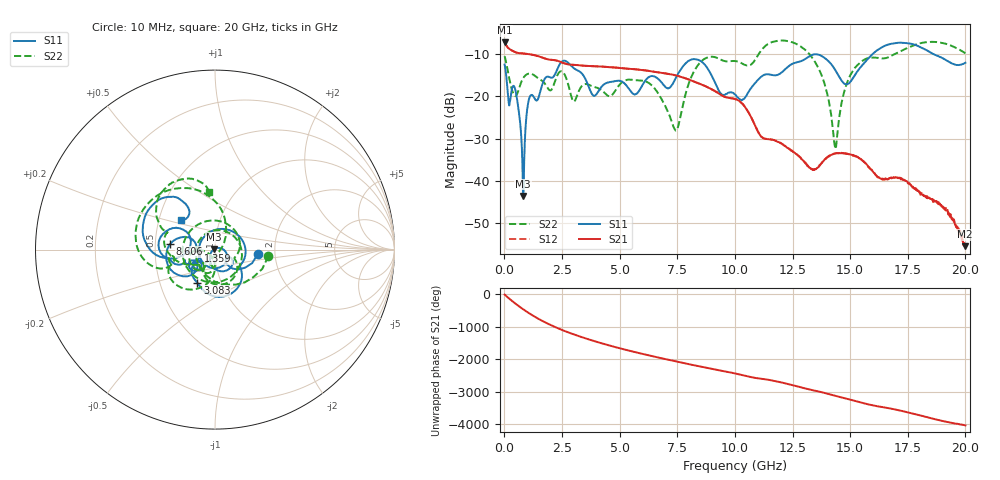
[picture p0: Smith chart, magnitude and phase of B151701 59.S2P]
!  2-Port S-parameters saved by WinCal
! VAR MeasName=S-Parameters (CALIBRATED_DATA) read from VNA (N5244A)
! VAR MeasDate=2015-12-24 19:16:58
! VAR NAME=B151701 59
! VAR FILENAME=B151701 59.S2P
! VAR DATE=2015-12-24 19:16:58
! VAR PHYS_PORTS=1,3
# Hz S DB R 50
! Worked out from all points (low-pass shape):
!   801 points, 10 MHz to 20 GHz, reference 50 ohm
!   highest |S21| = -7.16 dB at 10 MHz (marker M1); lowest = -55.4 dB at 19.98 GHz (marker M2)
!   |S21| within 3 dB of the highest: start of sweep to 1.25 GHz
!   lowest |S11| = -43.6 dB at 809.6 MHz (marker M3), VSWR 1.01, Z = 49.4 + j0.178 ohm
!   |S11| at or under -10 dB: start of sweep to 15.97 GHz; 18.63 GHz to end of sweep
!   |S22| runs from -32.4 to -6.7 dB; largest |S21 - S12| = 0.0023
!   S11 on the Smith chart (normalised r, x): 10 MHz: 1.62, -0.09; 1.359 GHz: 0.83, -0.02; 3.083 GHz: 0.77, -0.30; 8.606 GHz: 0.60, +0.04; 20 GHz: 0.65, +0.22
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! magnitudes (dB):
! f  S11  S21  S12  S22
! 10 MHz  -12.4  -7.2  -7.1  -10.5
! 509.8 MHz  -19.3  -9.6  -9.6  -19.8
! 809.6 MHz  -43.6  -9.8  -9.8  -15.7
! 1.059 GHz  -20.8  -10.0  -10.0  -14.6
! 1.359 GHz  -20.9  -10.3  -10.3  -15.2
! 2.509 GHz  -11.7  -12.0  -12.0  -14.1
! 3.083 GHz  -13.6  -12.5  -12.5  -20.8
! 3.358 GHz  -14.5  -12.7  -12.7  -17.5
! 3.908 GHz  -19.8  -12.8  -12.8  -17.8
! 6.682 GHz  -15.9  -14.3  -14.3  -19.3
! 7.456 GHz  -15.4  -15.0  -15.0  -28.0
! 8.606 GHz  -12.0  -17.3  -17.3  -11.4
! 10.01 GHz  -19.5  -20.6  -20.6  -11.6
! 11.98 GHz  -14.5  -31.0  -31.0  -6.8
! 13.35 GHz  -10.2  -37.2  -37.2  -10.8
! 13.93 GHz  -11.0  -34.8  -34.8  -17.7
! 14.35 GHz  -13.7  -33.4  -33.4  -32.1
! 15.1 GHz  -15.8  -33.9  -33.8  -14.0
! 16.68 GHz  -7.7  -39.3  -39.3  -10.7
! 18.9 GHz  -10.6  -45.4  -45.5  -7.3
! 19.98 GHz  -12.1  -55.4  -55.3  -9.7
! 20 GHz  -12.0  -55.0  -55.2  -9.8
